{attribute 'linkalways'}
VAR_GLOBAL
	// EL1008通道1
	bIBTN01  AT %I* : BOOL;
	// EL1008通道2
	bIBTN02  AT %I* : BOOL;
	// EL1008通道3
	bIBTN03  AT %I* : BOOL;
	// EL1008通道4
	bIBTN04  AT %I* : BOOL;
	// EL1008通道5
	bIBTN05  AT %I* : BOOL;
	// EL1008通道6
	bIBTN06  AT %I* : BOOL;
	// EL1008通道7
	bIBTN07  AT %I* : BOOL;
	// EL1008通道8
	bIBTN08  AT %I* : BOOL;

END_VAR
